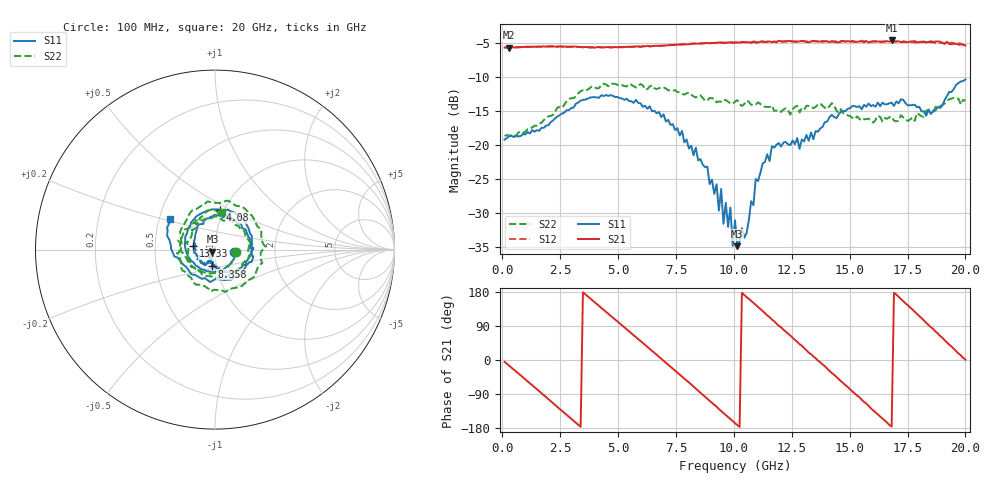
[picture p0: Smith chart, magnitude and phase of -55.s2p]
!Agilent Technologies,N5230C,MY49001569,A.09.33.09
!Agilent N5230C: A.09.33.09
!Date: Thursday, July 23, 2015 16:43:41
!Correction: S11(Full 2 Port(1,2))
!S21(Full 2 Port(1,2))
!S12(Full 2 Port(1,2))
!S22(Full 2 Port(1,2))
!S2P File: Measurements: S11, S21, S12, S22:
# Hz S  dB  R 50
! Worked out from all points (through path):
!   201 points, 100 MHz to 20 GHz, reference 50 ohm
!   highest |S21| = -4.62 dB at 16.82 GHz (marker M1); lowest = -5.7 dB at 299 MHz (marker M2)
!   group delay of S21, straight-line fit = 149 ps
!   lowest |S11| = -34.9 dB at 10.15 GHz (marker M3), VSWR 1.04, Z = 48.6 - j1.07 ohm
!   |S11| at or under -10 dB: start of sweep to end of sweep
!   |S22| runs from -18.7 to -11.0 dB; largest |S21 - S12| = 0.02
!   S11 on the Smith chart (normalised r, x): 100 MHz: 1.24, -0.04; 4.08 GHz: 0.96, +0.45; 8.358 GHz: 0.95, -0.18; 13.33 GHz: 0.78, +0.03; 20 GHz: 0.57, +0.22
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1e8  -19.21 -8.3  -5.66 -5.0  -5.65 -5.0  -18.67 -7.7
2.99e8  -18.72 -21.9  -5.70 -15.1  -5.68 -15.2  -18.62 -23.5
1.7915e9  -17.48 -133.3  -5.49 -92.9  -5.51 -93.0  -16.33 -135.6
3.483e9  -13.36 113.2  -5.62 178.6  -5.61 178.6  -11.95 119.6
4.08e9  -12.99 82.3  -5.61 147.8  -5.58 147.7  -11.68 90.2
5.3735e9  -13.19 20.9  -5.56 81.0  -5.62 81.0  -11.39 28.1
6.7665e9  -15.14 -41.3  -5.43 8.5  -5.39 8.3  -11.65 -30.1
8.3585e9  -20.39 -101.7  -5.07 -75.7  -5.10 -75.5  -13.01 -91.2
9.453e9  -26.46 -155.5  -4.94 -134.7  -4.93 -134.3  -13.62 -144.3
9.5525e9  -31.58 -147.4  -4.95 -139.7  -4.99 -139.6  -13.31 -147.2
9.851e9  -29.19 -175.3  -4.89 -155.9  -4.93 -155.6  -13.93 -161.5
9.9505e9  -34.83 -152.9  -4.95 -161.0  -4.93 -160.5  -13.92 -167.5
1.005e10  -31.05 171.9  -4.93 -166.8  -4.95 -166.7  -13.64 -173.8
1.01495e10  -34.87 -142.2  -4.90 -171.9  -4.97 -171.8  -13.40 -174.6
1.19405e10  -19.71 -121.9  -4.66 90.3  -4.86 91.2  -14.90 104.4
1.33335e10  -18.16 170.9  -4.78 15.4  -4.71 15.7  -14.40 29.4
1.3433e10  -19.14 167.3  -4.68 9.3  -4.74 10.7  -14.57 25.1
1.5224e10  -14.28 87.7  -4.83 -88.6  -4.78 -87.7  -16.16 -77.8
1.67165e10  -13.85 14.7  -4.81 -171.6  -4.76 -172.4  -15.92 -166.9
1.6816e10  -13.77 12.8  -4.62 -175.6  -4.79 -176.7  -15.83 -171.0
1.85075e10  -15.45 -110.3  -4.88 86.8  -4.70 87.7  -15.05 125.4
2e10  -10.35 145.6  -5.36 1.1  -5.34 1.2  -13.48 79.4
